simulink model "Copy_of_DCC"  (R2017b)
settings: Solver=FixedStepDiscrete  StartTime=0.0  StopTime=10.0  FixedStep=0.01  RelTol=1e-3  EnableMultiTasking=on
undefined symbols (not defined in the file): ASWTYPE_FALSE, ASWTYPE_TRUE, CbDCC_BMTMsgCmd_flg, CbDCC_BMVMsgCmd_flg, CbDCC_BSPMsgCmd_flg, CcDCC_BSTSendTi_ms, CcDCC_BulkSOC_pct, CcDCC_CCSTout_ms, CcDCC_CellTempFilterAvg_numb, CcDCC_ChrgCrnt0HysVolt_mV, CcDCC_ChrgFinOverTi_ms, CcDCC_ChrgMaxPackVoltLimt_V, CcDCC_ChrgSt2StepChrgTime_ms, CcDCC_ChrgStCutoffTime_ms, CcDCC_ChrgStFullChrgCrnt_A, CcDCC_CMLTout_ms, CcDCC_CommToutOverTi_ms, CcDCC_CRMAATout_ms, CcDCC_CRMCHMTout_ms, CcDCC_CRMTout_ms, CcDCC_CROAATout_ms, CcDCC_CROTout_ms, CcDCC_CSDTout_ms, CcDCC_CSTTout_ms, CcDCC_DC12VUnonnectTi_ms, CcDCC_DCChrgDispSOCPrmt_pct, CcDCC_DCChrgMismatch_ms, CcDCC_DCChrgPermitCfg_ms, CcDCC_DCChrgPrmtFltLvl_numb, CcDCC_DCChrgPrmtStop_ms, CcDCC_DCChrgStepCurr_A, CcDCC_DCChrgStop_ms, CcDCC_DCCrntUnctrolTi_ms, CcDCC_DCFullChrgHysVolt_mV, CcDCC_DCFullStepChrgTi1_ms, CcDCC_DCFullStepChrgTi2_ms, CcDCC_DCMaxChrgCurr_A, CcDCC_DCStepChrgWaitTime_ms, CcDCC_DCStop2DefaultTi_ms, CcDCC_DefaultWaitTi_ms, CcDCC_DiffDCChrgCrnt_A, CcDCC_DiffDCChrgCrntTi_ms, CcDCC_HeatChrgCrnt0Time_ms, CcDCC_HeatChrgCrnt1Time_ms, CcDCC_IsoDisableDelay_ms, CcDCC_MaxPackVoltLimt_V, CcDCC_SafeCur_A, CcDCC_StartChrgHysVolt_mV, CcDCC_StartDCChrgCellTemp_C, CcDCC_StepChrgCutoffTi_ms, CcDCC_StepChrgFullChrgCrnt_A, CcDCC_ToutDelay_ms, CcDCC_VehSpdFld_kmh, DCC_CONST0_NUMB, DCC_CONST1000_NUMB, DCC_CONST170_NUMB, DCC_RUNTIME_MS, Enum_BTMHeatReq, Enum_CTCCtrCtlConnMode, Enum_CTCCtrCtlState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
libraries: AIWAYS_Powertrain_BMS_lib x82
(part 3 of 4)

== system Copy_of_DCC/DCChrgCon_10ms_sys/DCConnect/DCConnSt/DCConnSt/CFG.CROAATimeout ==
  GbGDP_CRORecOnce_flg : Inport  OutDataTypeStr=boolean
  GbDCC_BROMsgCmd_flg : Inport  Port=2  OutDataTypeStr=boolean
  GcGDP_CROChrgrRdy_numb : Inport  Port=3  OutDataTypeStr=uint8
  GcDCS_2829Da_numb : Inport  Port=4  OutDataTypeStr=uint8
  CROAATimeout : TriggerPort  TriggerType=function-call  VariantControl=(inherit)  StatesWhenEnabling=reset
  Constant10 : Constant  Value=CcDCC_CROAATout_ms
  Constant11 : Constant  Value=DCC_CONST170_NUMB
  Constant12 : Constant  Value=DCC_CONST170_NUMB
  Constant8 : Constant  Value=ASWTYPE_TRUE
  Constant9 : Constant  Value=DCC_RUNTIME_MS
  Delay2 : AIWAYS_Powertrain_BMS_lib/Debounce & Delay/BMSDelay
  Logical Operator2 : Logic  Inputs=4  AllPortsSameDT=off  OutDataTypeStr=boolean
  Relational Operator3 : RelationalOperator  Operator===  OutDataTypeStr=boolean
  Relational Operator4 : RelationalOperator  Operator===  OutDataTypeStr=boolean
  Relational Operator5 : RelationalOperator  Operator=~=  OutDataTypeStr=boolean
  GbDCC_CROAATout_flg : Outport  OutDataTypeStr=boolean
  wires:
  GcDCS_2829Da_numb/1 -> Relational Operator4/1
  GcGDP_CROChrgrRdy_numb/1 -> Relational Operator5/1
  GbDCC_BROMsgCmd_flg/1 -> Logical Operator2/2
  GbGDP_CRORecOnce_flg/1 -> Relational Operator3/1
  Constant9/1 -> Delay2/2
  Constant11/1 -> Relational Operator5/2
  Constant12/1 -> Relational Operator4/2
  Constant10/1 -> Delay2/3
  Delay2/1 -> Logical Operator2/4
  Relational Operator5/1 -> Logical Operator2/3
  Constant8/1 -> Relational Operator3/2
  Relational Operator4/1 -> Delay2/1
  Relational Operator3/1 -> Logical Operator2/1
  Logical Operator2/1 -> GbDCC_CROAATout_flg/1

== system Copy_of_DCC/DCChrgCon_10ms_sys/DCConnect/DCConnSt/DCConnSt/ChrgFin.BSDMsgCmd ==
  GbGDP_CSTRecOnce_flg : Inport  OutDataTypeStr=boolean
  GbDCC_CSTTout_flg : Inport  Port=2
  BSDMsgCmd : TriggerPort  TriggerType=function-call  VariantControl=(inherit)  StatesWhenEnabling=reset
  Constant2 : Constant  Value=DCC_RUNTIME_MS
  Constant3 : Constant  Value=CcDCC_BSTSendTi_ms
  Delay : AIWAYS_Powertrain_BMS_lib/Debounce & Delay/BMSDelay
  Logical Operator : Logic  Operator=OR  AllPortsSameDT=off  OutDataTypeStr=boolean
  GbDCC_BSDMsgCmd_flg : Outport  OutDataTypeStr=boolean
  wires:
  Logical Operator/1 -> GbDCC_BSDMsgCmd_flg/1
  GbDCC_CSTTout_flg/1 -> Logical Operator/2
  Delay/1 -> Logical Operator/1
  Constant2/1 -> Delay/2
  Constant3/1 -> Delay/3
  GbGDP_CSTRecOnce_flg/1 -> Delay/1

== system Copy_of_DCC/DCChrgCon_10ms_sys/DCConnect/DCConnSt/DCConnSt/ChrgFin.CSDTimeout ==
  GbGDP_CSDRecOnce_flg : Inport  OutDataTypeStr=boolean
  CSDTimeout : TriggerPort  TriggerType=function-call  VariantControl=(inherit)  StatesWhenEnabling=reset
  Constant : Constant  Value=ASWTYPE_TRUE
  Constant2 : Constant  Value=DCC_RUNTIME_MS
  Constant3 : Constant  Value=CcDCC_CSDTout_ms
  Constant4 : Constant  Value=ASWTYPE_FALSE
  Delay : AIWAYS_Powertrain_BMS_lib/Debounce & Delay/BMSDelay
  Logical Operator : Logic  AllPortsSameDT=off  OutDataTypeStr=boolean
  Relational Operator1 : RelationalOperator  Operator===  OutDataTypeStr=boolean
  GbDCC_CSDTout_flg : Outport  OutDataTypeStr=boolean
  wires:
  Logical Operator/1 -> GbDCC_CSDTout_flg/1
  GbGDP_CSDRecOnce_flg/1 -> Relational Operator1/1
  Constant2/1 -> Delay/2
  Constant3/1 -> Delay/3
  Relational Operator1/1 -> Logical Operator/1
  Constant/1 -> Delay/1
  Delay/1 -> Logical Operator/2
  Constant4/1 -> Relational Operator1/2

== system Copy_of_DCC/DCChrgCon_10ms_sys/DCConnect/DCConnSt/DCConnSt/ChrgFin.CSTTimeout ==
  GbGDP_CSTRecOnce_flg : Inport  OutDataTypeStr=boolean
  CSTTimeout : TriggerPort  TriggerType=function-call  VariantControl=(inherit)  StatesWhenEnabling=reset
  Constant : Constant  Value=ASWTYPE_TRUE
  Constant2 : Constant  Value=DCC_RUNTIME_MS
  Constant3 : Constant  Value=CcDCC_CSTTout_ms
  Constant4 : Constant  Value=ASWTYPE_FALSE
  Delay : AIWAYS_Powertrain_BMS_lib/Debounce & Delay/BMSDelay
  Logical Operator : Logic  AllPortsSameDT=off  OutDataTypeStr=boolean
  Relational Operator1 : RelationalOperator  Operator===  OutDataTypeStr=boolean
  GbDCC_CSTTout_flg : Outport  OutDataTypeStr=boolean
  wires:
  Logical Operator/1 -> GbDCC_CSTTout_flg/1
  Constant4/1 -> Relational Operator1/2
  Constant3/1 -> Delay/3
  Constant2/1 -> Delay/2
  Constant/1 -> Delay/1
  Delay/1 -> Logical Operator/2
  Relational Operator1/1 -> Logical Operator/1
  GbGDP_CSTRecOnce_flg/1 -> Relational Operator1/1

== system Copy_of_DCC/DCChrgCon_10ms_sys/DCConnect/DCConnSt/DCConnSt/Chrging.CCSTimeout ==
  GbGDP_CCSMsgUpd_flg : Inport  OutDataTypeStr=boolean
  CCSTimeout : TriggerPort  TriggerType=function-call  VariantControl=(inherit)  StatesWhenEnabling=reset
  Constant2 : Constant  Value=DCC_RUNTIME_MS
  Constant3 : Constant  Value=CcDCC_CCSTout_ms
  Constant4 : Constant  Value=ASWTYPE_FALSE
  Delay : AIWAYS_Powertrain_BMS_lib/Debounce & Delay/BMSDelay
  Relational Operator : RelationalOperator  Operator===  OutDataTypeStr=boolean
  GbDCC_CCSTout_flg : Outport  OutDataTypeStr=boolean
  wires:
  Delay/1 -> GbDCC_CCSTout_flg/1
  Constant2/1 -> Delay/2
  GbGDP_CCSMsgUpd_flg/1 -> Relational Operator/1
  Constant4/1 -> Relational Operator/2
  Relational Operator/1 -> Delay/1
  Constant3/1 -> Delay/3

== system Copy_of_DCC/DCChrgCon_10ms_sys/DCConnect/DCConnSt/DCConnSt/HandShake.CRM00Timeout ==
  GbGDP_CHMRecOnce_flg : Inport  OutDataTypeStr=boolean
  CRM00Timeout : TriggerPort  TriggerType=function-call  VariantControl=(inherit)  StatesWhenEnabling=reset
  Constant : Constant  Value=ASWTYPE_TRUE
  Constant2 : Constant  Value=DCC_RUNTIME_MS
  Constant3 : Constant  Value=CcDCC_CRMTout_ms
  Constant5 : Constant  Value=DCC_RUNTIME_MS
  Constant6 : Constant  Value=CcDCC_CRMCHMTout_ms
  Constant7 : Constant  Value=ASWTYPE_TRUE
  Delay : AIWAYS_Powertrain_BMS_lib/Debounce & Delay/BMSDelay
  Delay1 : AIWAYS_Powertrain_BMS_lib/Debounce & Delay/BMSDelay
  Logical Operator2 : Logic  Operator=OR  AllPortsSameDT=off  OutDataTypeStr=boolean
  Relational Operator1 : RelationalOperator  Operator===  OutDataTypeStr=boolean
  GbDCC_CRM00Tout_flg : Outport  OutDataTypeStr=boolean
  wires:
  Delay/1 -> Logical Operator2/1
  Constant3/1 -> Delay/3
  Constant/1 -> Delay/1
  Constant2/1 -> Delay/2
  Constant7/1 -> Relational Operator1/2
  Constant6/1 -> Delay1/3
  GbGDP_CHMRecOnce_flg/1 -> Relational Operator1/1
  Constant5/1 -> Delay1/2
  Relational Operator1/1 -> Delay1/1
  Logical Operator2/1 -> GbDCC_CRM00Tout_flg/1
  Delay1/1 -> Logical Operator2/2

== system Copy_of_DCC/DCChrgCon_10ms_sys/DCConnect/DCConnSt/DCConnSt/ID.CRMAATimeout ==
  GbGDP_CRMRecOnce_flg : Inport  OutDataTypeStr=boolean
  GcGDP_CRMChrgrAck_numb : Inport  Port=2  OutDataTypeStr=uint8
  CRMAATimeout : TriggerPort  TriggerType=function-call  VariantControl=(inherit)  StatesWhenEnabling=reset
  Constant : Constant  Value=ASWTYPE_TRUE
  Constant1 : Constant  Value=ASWTYPE_TRUE
  Constant2 : Constant  Value=DCC_RUNTIME_MS
  Constant3 : Constant  Value=CcDCC_CRMAATout_ms
  Constant6 : Constant  Value=DCC_CONST170_NUMB
  Delay : AIWAYS_Powertrain_BMS_lib/Debounce & Delay/BMSDelay
  Logical Operator : Logic  Inputs=3  AllPortsSameDT=off  OutDataTypeStr=boolean
  Relational Operator : RelationalOperator  Operator===  OutDataTypeStr=boolean
  Relational Operator1 : RelationalOperator  Operator=~=  OutDataTypeStr=boolean
  GbDCC_CRMAATout_flg : Outport  OutDataTypeStr=boolean
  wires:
  Logical Operator/1 -> GbDCC_CRMAATout_flg/1
  Delay/1 -> Logical Operator/3
  Constant6/1 -> Relational Operator1/2
  Constant3/1 -> Delay/3
  Constant1/1 -> Relational Operator/2
  Relational Operator1/1 -> Logical Operator/2
  Relational Operator/1 -> Logical Operator/1
  GcGDP_CRMChrgrAck_numb/1 -> Relational Operator1/1
  Constant2/1 -> Delay/2
  GbGDP_CRMRecOnce_flg/1 -> Relational Operator/1
  Constant/1 -> Delay/1

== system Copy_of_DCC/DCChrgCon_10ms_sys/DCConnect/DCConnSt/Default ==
  GeLDP_CC2St_enum : Inport
  GbLDP_DC12VSply_flg : Inport  Port=2
  GcADP_VehSpd_kmh : Inport  Port=3
  Enable : EnablePort  StatesWhenEnabling=reset
  Constant : Constant  Value=Enum_LDPCC2St.Enum_LDPCC2St_Connect
  Constant1 : Constant  Value=ASWTYPE_TRUE
  Constant10 : Constant  Value=CcDCC_DefaultWaitTi_ms
  Constant5 : Constant  Value=CcDCC_VehSpdFld_kmh
  Constant9 : Constant  Value=DCC_RUNTIME_MS
  Data Type Conversion2 : DataTypeConversion
  Delay : AIWAYS_Powertrain_BMS_lib/Debounce & Delay/BMSDelay
  Logical Operator : Logic  Inputs=3  AllPortsSameDT=off  OutDataTypeStr=boolean
  Relational Operator1 : RelationalOperator  Operator===  OutDataTypeStr=boolean
  Relational Operator5 : RelationalOperator  Operator=<  OutDataTypeStr=boolean
  Relational Operator6 : RelationalOperator  Operator===  OutDataTypeStr=boolean
  LbDCC_DCDefault2Handshake_flg : Outport
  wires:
  Constant10/1 -> Delay/3
  Constant9/1 -> Delay/2
  Data Type Conversion2/1 -> Relational Operator6/1
  Constant/1 -> Relational Operator6/2
  GeLDP_CC2St_enum/1 -> Data Type Conversion2/1
  GbLDP_DC12VSply_flg/1 -> Relational Operator1/1
  Relational Operator5/1 -> Logical Operator/3
  Constant5/1 -> Relational Operator5/2
  GcADP_VehSpd_kmh/1 -> Relational Operator5/1
  Relational Operator1/1 -> Logical Operator/2
  Constant1/1 -> Relational Operator1/2
  Relational Operator6/1 -> Logical Operator/1
  Logical Operator/1 -> Delay/1
  Delay/1 -> LbDCC_DCDefault2Handshake_flg/1  "LbDCC_DCDefault2Handshake_flg"

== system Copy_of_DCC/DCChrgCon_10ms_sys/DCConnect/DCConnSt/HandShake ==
  GbLDP_DC12VSply_flg : Inport
  Enable : EnablePort  StatesWhenEnabling=reset
  Constant1 : Constant  Value=DCC_RUNTIME_MS
  Constant2 : Constant  Value=ASWTYPE_FALSE
  Constant5 : Constant  Value=CcDCC_DC12VUnonnectTi_ms
  Delay1 : AIWAYS_Powertrain_BMS_lib/Debounce & Delay/BMSDelay
  Relational Operator1 : RelationalOperator  Operator===  OutDataTypeStr=boolean
  LbDCC_DCHandShake2Default_flg : Outport
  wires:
  Constant1/1 -> Delay1/2
  Constant5/1 -> Delay1/3
  Relational Operator1/1 -> Delay1/1
  Delay1/1 -> LbDCC_DCHandShake2Default_flg/1  "LbDCC_DCHandShake2Default_flg"
  GbLDP_DC12VSply_flg/1 -> Relational Operator1/1
  Constant2/1 -> Relational Operator1/2

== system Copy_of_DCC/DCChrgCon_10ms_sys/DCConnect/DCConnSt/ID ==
  GbLDP_DC12VSply_flg : Inport
  Enable : EnablePort  StatesWhenEnabling=reset
  Constant1 : Constant  Value=DCC_RUNTIME_MS
  Constant2 : Constant  Value=ASWTYPE_FALSE
  Constant5 : Constant  Value=CcDCC_DC12VUnonnectTi_ms
  Delay1 : AIWAYS_Powertrain_BMS_lib/Debounce & Delay/BMSDelay
  Relational Operator1 : RelationalOperator  Operator===  OutDataTypeStr=boolean
  LbDCC_DCID2Default_flg : Outport
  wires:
  Constant1/1 -> Delay1/2
  Constant5/1 -> Delay1/3
  Relational Operator1/1 -> Delay1/1
  Delay1/1 -> LbDCC_DCID2Default_flg/1  "LbDCC_DCID2Default_flg"
  GbLDP_DC12VSply_flg/1 -> Relational Operator1/1
  Constant2/1 -> Relational Operator1/2

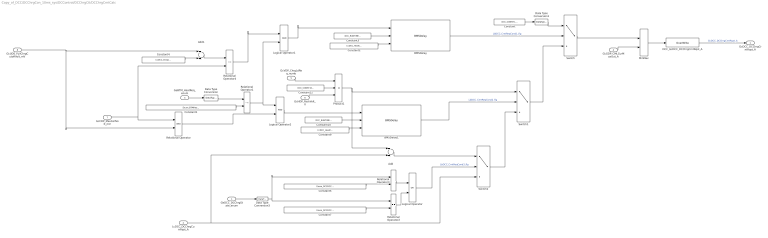
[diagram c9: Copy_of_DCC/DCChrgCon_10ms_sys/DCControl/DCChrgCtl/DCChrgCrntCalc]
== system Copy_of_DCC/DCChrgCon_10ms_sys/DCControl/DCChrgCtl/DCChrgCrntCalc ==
  GeDCC_DCChrgState_enum : Inport
  LcDCC_DCChrgCurrRqst_A : Inport  Port=2
  GeBTM_HeatReq_enum : Inport  Port=3
  GcGDP_CMLCurMaxOut_A : Inport  Port=4
  GcVDP_ChrgLdReq_numb : Inport  Port=5
  GcHDP_PackVolt_V : Inport  Port=6
  GcCDP_MaxCellVolt_mV : Inport  Port=7
  GcUDS_FullChrgCutoffVolt_mV : Inport  Port=8
  Add : Sum  OutDataTypeStr=single
  Add1 : Sum
  BMSDelay : AIWAYS_Powertrain_BMS_lib/Debounce & Delay/BMSDelay
  BMSDelay1 : AIWAYS_Powertrain_BMS_lib/Debounce & Delay/BMSDelay
  Constant : Constant  Value=DCC_CONST0_NUMB
  Constant1 : Constant  Value=Enum_BTMHeatReq.Enum_BTMHeatReq_Default
  Constant10 : Constant  Value=DCC_RUNTIME_MS
  Constant12 : Constant  Value=DCC_CONST1000_NUMB
  Constant2 : Constant  Value=CcDCC_HeatChrgCrnt0Time_ms
  Constant3 : Constant  Value=DCC_RUNTIME_MS
  Constant4 : Constant  Value=CcDCC_ChrgCrnt0HysVolt_mV
  Constant5 : Constant  Value=Enum_DCCDCChrgState.Enum_DCCDCChrgState_Chrg
  Constant7 : Constant  Value=Enum_DCCDCChrgState.Enum_DCCDCChrgState_StepChrg
  Constant9 : Constant  Value=CcDCC_HeatChrgCrnt1Time_ms
  DCC_GcDCC_DCChrgCrntRqst_A : AIWAYS_Powertrain_BMS_lib/Signals/OverWrite  OverWrite_Value=CcDCC_DCChrgCrntRqstOvr_A  OverWrite_flag=CbDCC_DCChrgCrntRqstOvrSwt_flg
  Data Type Conversion : DataTypeConversion
  Data Type Conversion1 : DataTypeConversion
  Data Type Conversion3 : DataTypeConversion
  Logical Operator : Logic  Operator=OR  AllPortsSameDT=off  OutDataTypeStr=boolean
  Logical Operator1 : Logic  AllPortsSameDT=off  OutDataTypeStr=boolean
  Logical Operator2 : Logic  AllPortsSameDT=off  OutDataTypeStr=boolean
  MinMax : MinMax  Inputs=2
  Product1 : Product  Inputs=**/  OutDataTypeStr=Inherit: Inherit via back propagation
  Relational Operator : RelationalOperator  OutDataTypeStr=boolean
  Relational Operator1 : RelationalOperator  Operator=~=  OutDataTypeStr=boolean
  Relational Operator2 : RelationalOperator  Operator===  OutDataTypeStr=boolean
  Relational Operator3 : RelationalOperator  Operator===  OutDataTypeStr=boolean
  Relational Operator4 : RelationalOperator  Operator=<=  OutDataTypeStr=boolean
  Switch : Switch  Criteria=u2 ~= 0  Threshold=1  RndMeth=Zero
  Switch1 : Switch  Criteria=u2 ~= 0  Threshold=1  RndMeth=Zero
  Switch2 : Switch  Criteria=u2 ~= 0  Threshold=1  RndMeth=Zero
  GcDCC_DCChrgCrntRqst_A : Outport
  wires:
  GcGDP_CMLCurMaxOut_A/1 -> MinMax/2
  Relational Operator2/1 -> Logical Operator/2
  Constant7/1 -> Relational Operator2/2
  Constant5/1 -> Relational Operator3/2
  Relational Operator3/1 -> Logical Operator/1
  GeDCC_DCChrgState_enum/1 -> Data Type Conversion3/1
  LcDCC_DCChrgCurrRqst_A/1 -> Add/2, Switch2/3
  Data Type Conversion3/1 -> Relational Operator3/1, Relational Operator2/1
  GcVDP_ChrgLdReq_numb/1 -> Product1/1
  Constant1/1 -> Relational Operator1/2
  GeBTM_HeatReq_enum/1 -> Data Type Conversion/1
  GcCDP_MaxCellVolt_mV/1 -> Relational Operator4/2, Relational Operator/1
  Constant2/1 -> BMSDelay/3
  Constant3/1 -> BMSDelay/2
  GcUDS_FullChrgCutoffVolt_mV/1 -> Relational Operator/2, Add1/1
  Constant4/1 -> Add1/2
  Add1/1 -> Relational Operator4/1
  Data Type Conversion/1 -> Relational Operator1/1
  Relational Operator4/1 -> Logical Operator1/1
  Relational Operator1/1 -> Logical Operator2/1, Logical Operator1/2
  Relational Operator/1 -> Logical Operator2/2
  Logical Operator1/1 -> BMSDelay/1
  Logical Operator2/1 -> BMSDelay1/1
  Constant10/1 -> BMSDelay1/2
  Constant9/1 -> BMSDelay1/3
  BMSDelay/1 -> Switch/2  "LbDCC_CrntReqCond1_flg"
  Constant/1 -> Data Type Conversion1/1
  BMSDelay1/1 -> Switch1/2  "LbDCC_CrntReqCond2_flg"
  Switch1/1 -> Switch/3
  Product1/1 -> Add/1, Switch1/1
  Logical Operator/1 -> Switch2/2  "LbDCC_CrntReqCond3_flg"
  Switch2/1 -> Switch1/3
  Add/1 -> Switch2/1
  GcHDP_PackVolt_V/1 -> Product1/3
  Constant12/1 -> Product1/2
  Switch/1 -> MinMax/1
  MinMax/1 -> DCC_GcDCC_DCChrgCrntRqst_A/1
  DCC_GcDCC_DCChrgCrntRqst_A/1 -> GcDCC_DCChrgCrntRqst_A/1  "GcDCC_DCChrgCrntRqst_A"
  Data Type Conversion1/1 -> Switch/1

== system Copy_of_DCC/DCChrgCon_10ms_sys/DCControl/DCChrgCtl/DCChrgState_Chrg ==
  GcDCC_DCChrgCrntRqst_A : Inport
  GcCDP_MaxCellVolt_mV : Inport  Port=2
  GeBTM_HeatReq_enum : Inport  Port=3
  GbDCC_DCChrgPrmt_flg : Inport  Port=4
  GeVDP_ChrgRqst_enum : Inport  Port=5
  GeDCC_DCConnSt_enum : Inport  Port=6
  GcUDS_FullChrgCutoffVolt_mV : Inport  Port=7
  Enable : EnablePort  StatesWhenEnabling=reset
  Bus Creator : BusCreator  Inputs=7
  Bus Selector : BusSelector  OutputSignals=GcDCC_DCChrgCrntRqst_A,GcCDP_MaxCellVolt_mV,GeBTM_HeatReq_enum,GcUDS_FullChrgCutoffVolt_mV
  Bus Selector1 : BusSelector  OutputSignals=GbDCC_DCChrgPrmt_flg,GcDCC_DCChrgCrntRqst_A,GcCDP_MaxCellVolt_mV,GeBTM_HeatReq_enum,GeVDP_ChrgRqst_enum,GeDCC_DCConnSt_enum,GcUDS_FullChrgCutoffVolt_mV
  Bus Selector2 : BusSelector  OutputSignals=GcCDP_MaxCellVolt_mV,GcUDS_FullChrgCutoffVolt_mV
  DCChrgCrntUnctrol : Subsystem
  DCChrgStateChrg2StepChrg : Subsystem
  DCChrgStateChrg2Stop : Subsystem
  LbDCC_ChrgSt2StepChrg_flg : Outport
  LbDCC_ChrgSt2Stop_flg : Outport  Port=2
  LbDCC_FinishInChrgSt_flg : Outport  Port=3
  GbDCC_DCCrntUnctrolFlt_flg : Outport  Port=4
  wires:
  DCChrgStateChrg2StepChrg/1(LbDCC_ChrgSt2StepChrg_flg) -> LbDCC_ChrgSt2StepChrg_flg/1
  DCChrgStateChrg2Stop/1(LbDCC_ChrgSt2Stop_flg) -> LbDCC_ChrgSt2Stop_flg/1
  DCChrgStateChrg2Stop/2(LbDCC_FinishInChrgSt_flg) -> LbDCC_FinishInChrgSt_flg/1
  GcDCC_DCChrgCrntRqst_A/1 -> Bus Creator/1
  GcCDP_MaxCellVolt_mV/1 -> Bus Creator/2
  GeBTM_HeatReq_enum/1 -> Bus Creator/3
  GbDCC_DCChrgPrmt_flg/1 -> Bus Creator/4
  GeVDP_ChrgRqst_enum/1 -> Bus Creator/5
  Bus Creator/1 -> Bus Selector/1, Bus Selector1/1, Bus Selector2/1
  Bus Selector/1 -> DCChrgStateChrg2StepChrg/1(GcDCC_DCChrgCrntRqst_A)  "<GcDCC_DCChrgCrntRqst_A>"
  Bus Selector/2 -> DCChrgStateChrg2StepChrg/2(GcCDP_MaxCellVolt_mV)  "<GcCDP_MaxCellVolt_mV>"
  Bus Selector/3 -> DCChrgStateChrg2StepChrg/3(GeBTM_HeatReq_enum)  "<GeBTM_HeatReq_enum>"
  Bus Selector1/1 -> DCChrgStateChrg2Stop/1(GbDCC_DCChrgPrmt_flg)  "<GbDCC_DCChrgPrmt_flg>"
  Bus Selector1/2 -> DCChrgStateChrg2Stop/2(GcDCC_DCChrgCrntRqst_A)  "<GcDCC_DCChrgCrntRqst_A>"
  Bus Selector1/3 -> DCChrgStateChrg2Stop/3(GcCDP_MaxCellVolt_mV)  "<GcCDP_MaxCellVolt_mV>"
  Bus Selector1/4 -> DCChrgStateChrg2Stop/4(GeBTM_HeatReq_enum)  "<GeBTM_HeatReq_enum>"
  DCChrgCrntUnctrol/1(GbDCC_DCCrntUnctrolFlt_flg) -> DCChrgStateChrg2Stop/8(GbDCC_DCCrntUnctrolFlt_flg), GbDCC_DCCrntUnctrolFlt_flg/1
  Bus Selector1/5 -> DCChrgStateChrg2Stop/5(GeVDP_ChrgRqst_enum)  "<GeVDP_ChrgRqst_enum>"
  Bus Selector2/1 -> DCChrgCrntUnctrol/1(GcCDP_MaxCellVolt_mV)  "<GcCDP_MaxCellVolt_mV>"
  GeDCC_DCConnSt_enum/1 -> Bus Creator/6
  Bus Selector1/6 -> DCChrgStateChrg2Stop/6(GeDCC_DCConnSt_enum)  "<GeDCC_DCConnSt_enum>"
  GcUDS_FullChrgCutoffVolt_mV/1 -> Bus Creator/7
  Bus Selector/4 -> DCChrgStateChrg2StepChrg/4(GcUDS_FullChrgCutoffVolt_mV)  "<GcUDS_FullChrgCutoffVolt_mV>"
  Bus Selector2/2 -> DCChrgCrntUnctrol/2(GcUDS_FullChrgCutoffVolt_mV)  "<GcUDS_FullChrgCutoffVolt_mV>"
  Bus Selector1/7 -> DCChrgStateChrg2Stop/7(GcUDS_FullChrgCutoffVolt_mV)  "<GcUDS_FullChrgCutoffVolt_mV>"

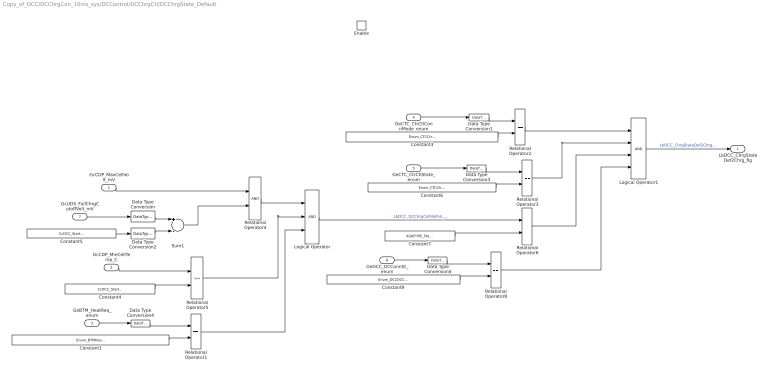
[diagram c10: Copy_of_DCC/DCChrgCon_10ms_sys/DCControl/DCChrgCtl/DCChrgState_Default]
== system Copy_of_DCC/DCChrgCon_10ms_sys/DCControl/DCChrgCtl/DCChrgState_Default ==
  GcCDP_MaxCellVolt_mV : Inport
  GcCDP_MinCellTemp_C : Inport  Port=2
  GeBTM_HeatReq_enum : Inport  Port=3
  GeCTC_CtrCtlConnMode_enum : Inport  Port=4
  GeCTC_CtrCtlState_enum : Inport  Port=5
  GeDCC_DCConnSt_enum : Inport  Port=6
  GcUDS_FullChrgCutoffVolt_mV : Inport  Port=7
  Enable : EnablePort  StatesWhenEnabling=reset
  Constant1 : Constant  Value=Enum_BTMHeatReq.Enum_BTMHeatReq_Default
  Constant3 : Constant  Value=Enum_CTCCtrCtlConnMode.Enum_CTCCtrCtlConnMode_DCChrg
  Constant4 : Constant  Value=CcDCC_StartDCChrgCellTemp_C
  Constant5 : Constant  Value=CcDCC_StartChrgHysVolt_mV
  Constant6 : Constant  Value=Enum_CTCCtrCtlState.Enum_CTCCtrCtlState_Online
  Constant7 : Constant  Value=ASWTYPE_FALSE
  Constant9 : Constant  Value=Enum_DCCDCConnSt.Enum_DCCDCConnSt_Chrging
  Data Type Conversion : DataTypeConversion  OutDataTypeStr=single
  Data Type Conversion{1,3..5} (4 alike) : DataTypeConversion
  Data Type Conversion2 : DataTypeConversion  OutDataTypeStr=single
  Logical Operator : Logic  Inputs=3  AllPortsSameDT=off  OutDataTypeStr=boolean
  Logical Operator1 : Logic  Inputs=4  AllPortsSameDT=off  OutDataTypeStr=boolean
  Relational Operator{1..3,6,8} (5 alike) : RelationalOperator  Operator===  OutDataTypeStr=boolean
  Relational Operator4 : RelationalOperator  OutDataTypeStr=boolean
  Relational Operator5 : RelationalOperator  Operator=<=  OutDataTypeStr=boolean
  Sum1 : Sum  Inputs=+-  OutDataTypeStr=Inherit: Inherit via back propagation  RndMeth=Zero
  LbDCC_ChrgStateDef2Chrg_flg : Outport
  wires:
  GcCDP_MaxCellVolt_mV/1 -> Relational Operator4/1
  Logical Operator/1 -> Relational Operator6/1  "LbDCC_DCChrgCellVoltHi_flg"
  Relational Operator4/1 -> Logical Operator/1
  Relational Operator5/1 -> Logical Operator/2
  Constant1/1 -> Relational Operator1/2
  GeBTM_HeatReq_enum/1 -> Data Type Conversion4/1
  Data Type Conversion4/1 -> Relational Operator1/1
  GcCDP_MinCellTemp_C/1 -> Relational Operator5/1
  GcUDS_FullChrgCutoffVolt_mV/1 -> Data Type Conversion/1
  Constant4/1 -> Relational Operator5/2
  Sum1/1 -> Relational Operator4/2
  Relational Operator1/1 -> Logical Operator/3
  Constant5/1 -> Data Type Conversion2/1
  GeCTC_CtrCtlConnMode_enum/1 -> Data Type Conversion1/1
  Logical Operator1/1 -> LbDCC_ChrgStateDef2Chrg_flg/1  "LbDCC_ChrgStateDef2Chrg_flg"
  Constant7/1 -> Relational Operator6/2
  Relational Operator6/1 -> Logical Operator1/3
  Relational Operator3/1 -> Logical Operator1/2
  Constant3/1 -> Relational Operator2/2
  Data Type Conversion3/1 -> Relational Operator3/1
  Data Type Conversion1/1 -> Relational Operator2/1
  Constant6/1 -> Relational Operator3/2
  GeCTC_CtrCtlState_enum/1 -> Data Type Conversion3/1
  Data Type Conversion/1 -> Sum1/1
  Data Type Conversion2/1 -> Sum1/2
  Relational Operator2/1 -> Logical Operator1/1
  Constant9/1 -> Relational Operator8/2
  GeDCC_DCConnSt_enum/1 -> Data Type Conversion5/1
  Data Type Conversion5/1 -> Relational Operator8/1
  Relational Operator8/1 -> Logical Operator1/4

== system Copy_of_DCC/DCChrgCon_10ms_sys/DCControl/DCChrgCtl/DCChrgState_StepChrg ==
  GcDCC_DCChrgCrntRqst_A : Inport
  GcCDP_MaxCellVolt_mV : Inport  Port=2
  GbDCC_DCChrgPrmt_flg : Inport  Port=3
  GeVDP_ChrgRqst_enum : Inport  Port=4
  GeDCC_DCConnSt_enum : Inport  Port=5
  GcUDS_FullChrgCutoffVolt_mV : Inport  Port=6
  Enable : EnablePort  StatesWhenEnabling=reset
  DCCrntInStepChrgRequest : Subsystem
  DCCurrentDecrease : Subsystem
  DCFullChrg : Subsystem
  DCStepChrg2Stop : Subsystem
  LcDCC_StepChrgCrntReq_A : Outport
  LbDCC_StepChrg2Stop_flg : Outport  Port=2
  LbDCC_FinishInStepChrg_flg : Outport  Port=3
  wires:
  GcDCC_DCChrgCrntRqst_A/1 -> DCCurrentDecrease/1(GcDCC_DCChrgCrntRqst_A)
  GcCDP_MaxCellVolt_mV/1 -> DCFullChrg/3(GcCDP_MaxCellVolt_mV), DCCurrentDecrease/2(GcCDP_MaxCellVolt_mV)
  GbDCC_DCChrgPrmt_flg/1 -> DCStepChrg2Stop/2(GbDCC_DCChrgPrmt_flg)
  DCCurrentDecrease/1(LbDCC_StepChrgVoltReach_flg) -> DCCrntInStepChrgRequest/1(LbDCC_StepChrgVoltReach_flg)
  DCCurrentDecrease/2(LcDCC_StepChrgCrntDec_A) -> DCCrntInStepChrgRequest/2(LcDCC_StepChrgCrntDec_A)
  DCCrntInStepChrgRequest/1(LcDCC_StepChrgCrntReq_A) -> DCFullChrg/1(LcDCC_StepChrgCrntReq_A), LcDCC_StepChrgCrntReq_A/1
  DCFullChrg/1(LbDCC_FinishInStepChrg_flg) -> LbDCC_FinishInStepChrg_flg/1, DCStepChrg2Stop/1(LbDCC_FinishInStepChrg_flg)
  DCStepChrg2Stop/1(LbDCC_StepChrg2Stop_flg) -> LbDCC_StepChrg2Stop_flg/1
  GeVDP_ChrgRqst_enum/1 -> DCStepChrg2Stop/3(GeVDP_ChrgRqst_enum)
  GeDCC_DCConnSt_enum/1 -> DCStepChrg2Stop/4(GeDCC_DCConnSt_enum)
  GcUDS_FullChrgCutoffVolt_mV/1 -> DCCurrentDecrease/3(GcUDS_FullChrgCutoffVolt_mV), DCFullChrg/2(GcUDS_FullChrgCutoffVolt_mV)

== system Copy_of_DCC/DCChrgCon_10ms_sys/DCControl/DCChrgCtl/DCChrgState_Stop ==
  GeDCC_DCConnSt_enum : Inport
  Enable : EnablePort  StatesWhenEnabling=reset
  BMSDelay : AIWAYS_Powertrain_BMS_lib/Debounce & Delay/BMSDelay
  Constant : Constant  Value=ASWTYPE_TRUE
  Constant3 : Constant  Value=Enum_DCCDCConnSt.Enum_DCCDCConnSt_ID
  Constant4 : Constant  Value=CcDCC_DCStop2DefaultTi_ms
  Constant5 : Constant  Value=DCC_RUNTIME_MS
  Data Type Conversion5 : DataTypeConversion
  EdgeRising : AIWAYS_Powertrain_BMS_lib/Logical Operators/EdgeRising
  Logical1 : Logic  Operator=OR  OutDataTypeStr=boolean
  Relational Operator8 : RelationalOperator  Operator===  OutDataTypeStr=boolean
  LbDCC_Stop2Default_flg : Outport
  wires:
  Constant4/1 -> BMSDelay/3
  Constant5/1 -> BMSDelay/2
  Constant/1 -> BMSDelay/1
  Data Type Conversion5/1 -> Relational Operator8/1
  Constant3/1 -> Relational Operator8/2
  GeDCC_DCConnSt_enum/1 -> Data Type Conversion5/1
  Relational Operator8/1 -> EdgeRising/1
  BMSDelay/1 -> Logical1/1
  EdgeRising/1 -> Logical1/2
  Logical1/1 -> LbDCC_Stop2Default_flg/1  "LbDCC_Stop2Default_flg"

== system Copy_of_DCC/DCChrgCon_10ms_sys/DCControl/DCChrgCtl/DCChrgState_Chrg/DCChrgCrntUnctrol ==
  GcCDP_MaxCellVolt_mV : Inport
  GcUDS_FullChrgCutoffVolt_mV : Inport  Port=2
  Add : Sum
  BMSDebounceStartZero : AIWAYS_Powertrain_BMS_lib/Debounce & Delay/BMSDebounceStartZero
  Constant10 : Constant  Value=CcDCC_DCFullChrgHysVolt_mV
  Constant2 : Constant  Value=DCC_RUNTIME_MS
  Constant3 : Constant  Value=CcDCC_DCCrntUnctrolTi_ms
  Constant7 : Constant  Value=DCC_RUNTIME_MS
  Constant9 : Constant  Value=CcDCC_DCCrntUnctrolTi_ms
  DCC_GbDCC_DCCrntUnctrolFlt_flg : AIWAYS_Powertrain_BMS_lib/Signals/OverWrite  OverWrite_Value=CbDCC_DCCrntUnctrolFltOvr_flg  OverWrite_flag=CbDCC_DCCrntUnctrolFltOvrSwt_flg
  Relational Operator4 : RelationalOperator  OutDataTypeStr=boolean
  GbDCC_DCCrntUnctrolFlt_flg : Outport
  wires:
  GcCDP_MaxCellVolt_mV/1 -> Relational Operator4/1
  Add/1 -> Relational Operator4/2
  Constant10/1 -> Add/2
  Constant9/1 -> BMSDebounceStartZero/4
  Constant7/1 -> BMSDebounceStartZero/3
  GcUDS_FullChrgCutoffVolt_mV/1 -> Add/1
  Relational Operator4/1 -> BMSDebounceStartZero/1
  BMSDebounceStartZero/1 -> DCC_GbDCC_DCCrntUnctrolFlt_flg/1
  DCC_GbDCC_DCCrntUnctrolFlt_flg/1 -> GbDCC_DCCrntUnctrolFlt_flg/1  "GbDCC_DCCrntUnctrolFlt_flg"
  Constant2/1 -> BMSDebounceStartZero/5
  Constant3/1 -> BMSDebounceStartZero/2

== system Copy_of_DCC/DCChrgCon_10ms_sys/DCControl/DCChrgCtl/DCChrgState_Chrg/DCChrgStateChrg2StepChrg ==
  GcDCC_DCChrgCrntRqst_A : Inport
  GcCDP_MaxCellVolt_mV : Inport  Port=2
  GeBTM_HeatReq_enum : Inport  Port=3
  GcUDS_FullChrgCutoffVolt_mV : Inport  Port=4
  BMSDebounceStartZero : AIWAYS_Powertrain_BMS_lib/Debounce & Delay/BMSDebounceStartZero
  Constant1 : Constant  Value=CcDCC_ChrgSt2StepChrgTime_ms
  Constant2 : Constant  Value=DCC_RUNTIME_MS
  Constant3 : Constant  Value=Enum_BTMHeatReq.Enum_BTMHeatReq_Default
  Constant5 : Constant  Value=CcDCC_ChrgStFullChrgCrnt_A
  Constant6 : Constant  Value=DCC_RUNTIME_MS
  Constant7 : Constant  Value=CcDCC_ChrgSt2StepChrgTime_ms
  Data Type Conversion4 : DataTypeConversion
  Logical Operator : Logic  Inputs=3  AllPortsSameDT=off  OutDataTypeStr=boolean
  Relational Operator : RelationalOperator  OutDataTypeStr=boolean
  Relational Operator1 : RelationalOperator  Operator===  OutDataTypeStr=boolean
  Relational Operator3 : RelationalOperator  Operator=>  OutDataTypeStr=boolean
  LbDCC_ChrgSt2StepChrg_flg : Outport
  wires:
  GcCDP_MaxCellVolt_mV/1 -> Relational Operator/1
  Constant5/1 -> Relational Operator3/2
  Relational Operator3/1 -> Logical Operator/1
  GcUDS_FullChrgCutoffVolt_mV/1 -> Relational Operator/2
  Logical Operator/1 -> BMSDebounceStartZero/1
  Relational Operator/1 -> Logical Operator/2
  GcDCC_DCChrgCrntRqst_A/1 -> Relational Operator3/1
  Relational Operator1/1 -> Logical Operator/3
  Constant3/1 -> Relational Operator1/2
  GeBTM_HeatReq_enum/1 -> Data Type Conversion4/1
  Data Type Conversion4/1 -> Relational Operator1/1
  Constant2/1 -> BMSDebounceStartZero/3
  Constant1/1 -> BMSDebounceStartZero/4
  BMSDebounceStartZero/1 -> LbDCC_ChrgSt2StepChrg_flg/1  "LbDCC_ChrgSt2StepChrg_flg"
  Constant6/1 -> BMSDebounceStartZero/5
  Constant7/1 -> BMSDebounceStartZero/2

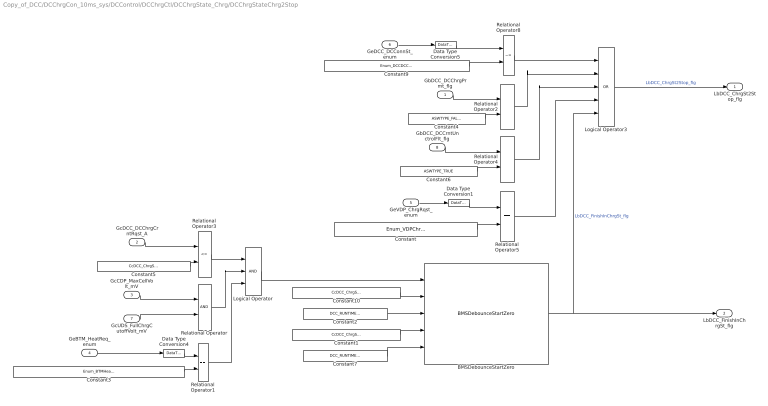
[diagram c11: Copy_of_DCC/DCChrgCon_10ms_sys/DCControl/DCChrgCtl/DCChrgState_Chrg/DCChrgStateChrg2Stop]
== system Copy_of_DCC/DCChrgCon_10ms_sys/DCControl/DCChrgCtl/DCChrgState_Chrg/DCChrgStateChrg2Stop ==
  GbDCC_DCChrgPrmt_flg : Inport
  GcDCC_DCChrgCrntRqst_A : Inport  Port=2
  GcCDP_MaxCellVolt_mV : Inport  Port=3
  GeBTM_HeatReq_enum : Inport  Port=4
  GeVDP_ChrgRqst_enum : Inport  Port=5
  GeDCC_DCConnSt_enum : Inport  Port=6
  GcUDS_FullChrgCutoffVolt_mV : Inport  Port=7
  GbDCC_DCCrntUnctrolFlt_flg : Inport  Port=8
  BMSDebounceStartZero : AIWAYS_Powertrain_BMS_lib/Debounce & Delay/BMSDebounceStartZero
  Constant : Constant  Value=Enum_VDPChrgRqst.Enum_VDPChrgRqst_PowerDown
  Constant1 : Constant  Value=CcDCC_ChrgStCutoffTime_ms
  Constant10 : Constant  Value=CcDCC_ChrgStCutoffTime_ms
  Constant2 : Constant  Value=DCC_RUNTIME_MS
  Constant3 : Constant  Value=Enum_BTMHeatReq.Enum_BTMHeatReq_Default
  Constant4 : Constant  Value=ASWTYPE_FALSE
  Constant5 : Constant  Value=CcDCC_ChrgStFullChrgCrnt_A
  Constant6 : Constant  Value=ASWTYPE_TRUE
  Constant7 : Constant  Value=DCC_RUNTIME_MS
  Constant9 : Constant  Value=Enum_DCCDCConnSt.Enum_DCCDCConnSt_Chrging
  Data Type Conversion1 : DataTypeConversion
  Data Type Conversion4 : DataTypeConversion
  Data Type Conversion5 : DataTypeConversion
  Logical Operator : Logic  Inputs=3  AllPortsSameDT=off  OutDataTypeStr=boolean
  Logical Operator3 : Logic  Operator=OR  Inputs=5  AllPortsSameDT=off  OutDataTypeStr=boolean
  Relational Operator : RelationalOperator  OutDataTypeStr=boolean
  Relational Operator{1..2,4..5} (4 alike) : RelationalOperator  Operator===  OutDataTypeStr=boolean
  Relational Operator3 : RelationalOperator  Operator=<=  OutDataTypeStr=boolean
  Relational Operator8 : RelationalOperator  Operator=~=  OutDataTypeStr=boolean
  LbDCC_ChrgSt2Stop_flg : Outport
  LbDCC_FinishInChrgSt_flg : Outport  Port=2
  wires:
  BMSDebounceStartZero/1 -> Logical Operator3/5, LbDCC_FinishInChrgSt_flg/1  "LbDCC_FinishInChrgSt_flg"
  Logical Operator3/1 -> LbDCC_ChrgSt2Stop_flg/1  "LbDCC_ChrgSt2Stop_flg"
  Constant4/1 -> Relational Operator2/2
  GbDCC_DCChrgPrmt_flg/1 -> Relational Operator2/1
  Constant1/1 -> BMSDebounceStartZero/4
  Constant5/1 -> Relational Operator3/2
  Relational Operator3/1 -> Logical Operator/1
  Logical Operator/1 -> BMSDebounceStartZero/1
  Relational Operator/1 -> Logical Operator/2
  GcDCC_DCChrgCrntRqst_A/1 -> Relational Operator3/1
  Constant3/1 -> Relational Operator1/2
  GeBTM_HeatReq_enum/1 -> Data Type Conversion4/1
  Data Type Conversion4/1 -> Relational Operator1/1
  Constant2/1 -> BMSDebounceStartZero/3
  GcCDP_MaxCellVolt_mV/1 -> Relational Operator/1
  Relational Operator1/1 -> Logical Operator/3
  GcUDS_FullChrgCutoffVolt_mV/1 -> Relational Operator/2
  Constant6/1 -> Relational Operator4/2
  GbDCC_DCCrntUnctrolFlt_flg/1 -> Relational Operator4/1
  Constant/1 -> Relational Operator5/2
  GeVDP_ChrgRqst_enum/1 -> Data Type Conversion1/1
  Data Type Conversion1/1 -> Relational Operator5/1
  GeDCC_DCConnSt_enum/1 -> Data Type Conversion5/1
  Constant9/1 -> Relational Operator8/2
  Data Type Conversion5/1 -> Relational Operator8/1
  Relational Operator8/1 -> Logical Operator3/1
  Relational Operator2/1 -> Logical Operator3/2
  Relational Operator4/1 -> Logical Operator3/3
  Relational Operator5/1 -> Logical Operator3/4
  Constant7/1 -> BMSDebounceStartZero/5
  Constant10/1 -> BMSDebounceStartZero/2

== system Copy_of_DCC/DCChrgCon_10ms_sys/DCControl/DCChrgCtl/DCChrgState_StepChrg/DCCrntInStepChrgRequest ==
  LbDCC_StepChrgVoltReach_flg : Inport  OutDataTypeStr=boolean
  LcDCC_StepChrgCrntDec_A : Inport  Port=2
  Constant : Constant  Value=DCC_CONST0_NUMB
  Data Type Conversion : DataTypeConversion
  Switch : Switch  Criteria=u2 ~= 0
  LcDCC_StepChrgCrntReq_A : Outport
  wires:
  LcDCC_StepChrgCrntDec_A/1 -> Switch/3
  Switch/1 -> LcDCC_StepChrgCrntReq_A/1  "LcDCC_StepChrgCrntReq_A"
  LbDCC_StepChrgVoltReach_flg/1 -> Switch/2
  Constant/1 -> Data Type Conversion/1
  Data Type Conversion/1 -> Switch/1

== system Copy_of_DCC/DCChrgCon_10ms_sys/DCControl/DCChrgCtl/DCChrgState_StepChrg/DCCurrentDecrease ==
  GcDCC_DCChrgCrntRqst_A : Inport
  GcCDP_MaxCellVolt_mV : Inport  Port=2
  GcUDS_FullChrgCutoffVolt_mV : Inport  Port=3
  BMSDebounceStartZero : AIWAYS_Powertrain_BMS_lib/Debounce & Delay/BMSDebounceStartZero
  Constant1 : Constant  Value=CcDCC_StepChrgCutoffTi_ms
  Constant2 : Constant  Value=DCC_RUNTIME_MS
  Constant4 : Constant  Value=ASWTYPE_FALSE
  Constant5 : Constant  Value=ASWTYPE_FALSE
  Constant6 : Constant  Value=DCC_RUNTIME_MS
  Constant7 : Constant  Value=CcDCC_StepChrgCutoffTi_ms
  DCStepChrgVoltReach : Subsystem  TreatAsAtomicUnit=on
  Logical Operator : Logic  Operator=OR  Inputs=3  AllPortsSameDT=off  OutDataTypeStr=boolean
  Relational Operator : RelationalOperator  OutDataTypeStr=boolean
  Subsystem : Subsystem
  Switch : Switch  Criteria=u2 ~= 0  Threshold=""
  Unit Delay : UnitDelay  InitialCondition=ASWTYPE_TRUE  SampleTime=-1  StateName=StateName
  Unit Delay External IC : AIWAYS_Powertrain_BMS_lib/Delay Blocks/Unit Delay External IC
  Unit Delay1 : UnitDelay  InitialCondition=ASWTYPE_FALSE  SampleTime=-1  StateName=StateName
  Unit Delay2 : UnitDelay  InitialCondition=ASWTYPE_FALSE  SampleTime=-1  StateName=StateName
  LbDCC_StepChrgVoltReach_flg : Outport
  LcDCC_StepChrgCrntDec_A : Outport  Port=2
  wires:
  Unit Delay/1 -> Logical Operator/3, Subsystem/Enable
  Switch/1 -> Logical Operator/1
  Unit Delay2/1 -> Switch/3
  Constant5/1 -> Switch/1
  Unit Delay1/1 -> Switch/2
  Logical Operator/1 -> LbDCC_StepChrgVoltReach_flg/1, DCStepChrgVoltReach/Enable, Unit Delay2/1  "LbDCC_StepChrgVoltReach_flg"
  Constant4/1 -> Unit Delay/1
  Relational Operator/1 -> BMSDebounceStartZero/1
  Constant1/1 -> BMSDebounceStartZero/4
  Constant2/1 -> BMSDebounceStartZero/3
  GcCDP_MaxCellVolt_mV/1 -> Relational Operator/1
  GcUDS_FullChrgCutoffVolt_mV/1 -> Relational Operator/2
  DCStepChrgVoltReach/1(LbDCC_DCStepWaitReach_flg) -> Unit Delay1/1
  Unit Delay External IC/1 -> DCStepChrgVoltReach/1(LcDCC_LastCrntRqst_A)  "LcDCC_LastCrntRqst_A"
  DCStepChrgVoltReach/2(LcDCC_StepChrgCrntDec_A) -> LcDCC_StepChrgCrntDec_A/1, Unit Delay External IC/1
  GcDCC_DCChrgCrntRqst_A/1 -> Subsystem/1(GcDCC_DCChrgCrntRqst_A)
  Subsystem/1(LcDCC_DCChrgCrntRqstLock_A) -> Unit Delay External IC/2
  BMSDebounceStartZero/1 -> Logical Operator/2
  Constant6/1 -> BMSDebounceStartZero/5
  Constant7/1 -> BMSDebounceStartZero/2

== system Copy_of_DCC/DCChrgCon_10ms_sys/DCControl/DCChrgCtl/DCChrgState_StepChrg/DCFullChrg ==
  LcDCC_StepChrgCrntReq_A : Inport
  GcUDS_FullChrgCutoffVolt_mV : Inport  Port=2
  GcCDP_MaxCellVolt_mV : Inport  Port=3
  Add : Sum
  BMSDebounceStartZero : AIWAYS_Powertrain_BMS_lib/Debounce & Delay/BMSDebounceStartZero
  BMSDebounceStartZero1 : AIWAYS_Powertrain_BMS_lib/Debounce & Delay/BMSDebounceStartZero
  Constant : Constant  Value=CcDCC_StepChrgFullChrgCrnt_A
  Constant1 : Constant  Value=CcDCC_DCFullStepChrgTi1_ms
  Constant{2,6,8,10} (4 alike) : Constant  Value=DCC_RUNTIME_MS
  Constant11 : Constant  Value=CcDCC_DCFullStepChrgTi2_ms
  Constant3 : Constant  Value=CcDCC_DCFullChrgHysVolt_mV
  Constant7 : Constant  Value=CcDCC_DCFullStepChrgTi2_ms
  Constant9 : Constant  Value=CcDCC_DCFullStepChrgTi1_ms
  Logical Operator1 : Logic  Operator=OR  AllPortsSameDT=off  OutDataTypeStr=boolean
  Logical Operator2 : Logic  AllPortsSameDT=off  OutDataTypeStr=boolean
  Relational Operator : RelationalOperator  Operator=<=  OutDataTypeStr=boolean
  Relational Operator1 : RelationalOperator  OutDataTypeStr=boolean
  Relational Operator2 : RelationalOperator  OutDataTypeStr=boolean
  LbDCC_FinishInStepChrg_flg : Outport
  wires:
  LcDCC_StepChrgCrntReq_A/1 -> Relational Operator/1
  Relational Operator1/1 -> BMSDebounceStartZero/1
  GcCDP_MaxCellVolt_mV/1 -> Relational Operator2/1, Relational Operator1/1
  Add/1 -> Relational Operator1/2
  Constant3/1 -> Add/2
  BMSDebounceStartZero/1 -> Logical Operator1/2
  Logical Operator1/1 -> LbDCC_FinishInStepChrg_flg/1  "LbDCC_FinishInStepChrg_flg"
  Constant/1 -> Relational Operator/2
  Constant2/1 -> BMSDebounceStartZero/3
  GcUDS_FullChrgCutoffVolt_mV/1 -> Relational Operator2/2, Add/1
  Relational Operator/1 -> Logical Operator2/1
  Relational Operator2/1 -> Logical Operator2/2
  Logical Operator2/1 -> BMSDebounceStartZero1/1
  BMSDebounceStartZero1/1 -> Logical Operator1/1
  Constant6/1 -> BMSDebounceStartZero1/3
  Constant1/1 -> BMSDebounceStartZero/4
  Constant8/1 -> BMSDebounceStartZero/5
  Constant9/1 -> BMSDebounceStartZero/2
  Constant7/1 -> BMSDebounceStartZero1/4
  Constant10/1 -> BMSDebounceStartZero1/5
  Constant11/1 -> BMSDebounceStartZero1/2

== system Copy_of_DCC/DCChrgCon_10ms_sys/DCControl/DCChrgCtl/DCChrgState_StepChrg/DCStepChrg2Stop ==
  LbDCC_FinishInStepChrg_flg : Inport
  GbDCC_DCChrgPrmt_flg : Inport  Port=2
  GeVDP_ChrgRqst_enum : Inport  Port=3
  GeDCC_DCConnSt_enum : Inport  Port=4
  Constant : Constant  Value=Enum_VDPChrgRqst.Enum_VDPChrgRqst_PowerDown
  Constant3 : Constant  Value=ASWTYPE_FALSE
  Constant9 : Constant  Value=Enum_DCCDCConnSt.Enum_DCCDCConnSt_Chrging
  Data Type Conversion1 : DataTypeConversion
  Data Type Conversion5 : DataTypeConversion
  Logical Operator1 : Logic  Operator=OR  Inputs=4  AllPortsSameDT=off  OutDataTypeStr=boolean
  Relational Operator1 : RelationalOperator  Operator===  OutDataTypeStr=boolean
  Relational Operator5 : RelationalOperator  Operator===  OutDataTypeStr=boolean
  Relational Operator8 : RelationalOperator  Operator=~=  OutDataTypeStr=boolean
  LbDCC_StepChrg2Stop_flg : Outport
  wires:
  GbDCC_DCChrgPrmt_flg/1 -> Relational Operator1/1
  Logical Operator1/1 -> LbDCC_StepChrg2Stop_flg/1  "LbDCC_StepChrg2Stop_flg"
  Relational Operator1/1 -> Logical Operator1/1
  Constant3/1 -> Relational Operator1/2
  LbDCC_FinishInStepChrg_flg/1 -> Logical Operator1/2
  GeVDP_ChrgRqst_enum/1 -> Data Type Conversion1/1
  Constant/1 -> Relational Operator5/2
  Data Type Conversion1/1 -> Relational Operator5/1
  Relational Operator5/1 -> Logical Operator1/3
  Constant9/1 -> Relational Operator8/2
  Data Type Conversion5/1 -> Relational Operator8/1
  GeDCC_DCConnSt_enum/1 -> Data Type Conversion5/1
  Relational Operator8/1 -> Logical Operator1/4

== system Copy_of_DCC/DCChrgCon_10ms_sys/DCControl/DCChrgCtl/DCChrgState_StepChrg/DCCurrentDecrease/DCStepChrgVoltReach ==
  LcDCC_LastCrntRqst_A : Inport
  Enable : EnablePort  StatesWhenEnabling=reset
  Add : Sum  Inputs=+-  AccumDataTypeStr=single  OutDataTypeStr=single
  BMSDelay : AIWAYS_Powertrain_BMS_lib/Debounce & Delay/BMSDelay
  Constant : Constant  Value=ASWTYPE_TRUE
  Constant2 : Constant  Value=DCC_RUNTIME_MS
  Constant3 : Constant  Value=CcDCC_DCChrgStepCurr_A
  Constant4 : Constant  Value=DCC_CONST0_NUMB
  Constant5 : Constant  Value=CcDCC_DCStepChrgWaitTime_ms
  Data Type Conversion : DataTypeConversion
  Limiter : AIWAYS_Powertrain_BMS_lib/Nonlinear Blocks/Limiter
  Switch : Switch  Criteria=u2 ~= 0
  LbDCC_DCStepWaitReach_flg : Outport
  LcDCC_StepChrgCrntDec_A : Outport  Port=2
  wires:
  BMSDelay/1 -> Switch/2, LbDCC_DCStepWaitReach_flg/1  "LbDCC_DCStepWaitReach_flg"
  LcDCC_LastCrntRqst_A/1 -> Limiter/1, Add/1, Switch/3
  Constant3/1 -> Add/2
  Add/1 -> Limiter/3
  Limiter/1 -> Switch/1
  Constant/1 -> BMSDelay/1
  Constant2/1 -> BMSDelay/2
  Constant5/1 -> BMSDelay/3
  Switch/1 -> LcDCC_StepChrgCrntDec_A/1  "LcDCC_StepChrgCrntDec_A"
  Constant4/1 -> Data Type Conversion/1
  Data Type Conversion/1 -> Limiter/2

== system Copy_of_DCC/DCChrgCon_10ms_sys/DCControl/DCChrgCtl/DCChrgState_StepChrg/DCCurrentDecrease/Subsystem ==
  GcDCC_DCChrgCrntRqst_A : Inport
  Enable : EnablePort
  Signal Conversion : SignalConversion  ConversionOutput=Contiguous copy  OverrideOpt=off
  LcDCC_DCChrgCrntRqstLock_A : Outport
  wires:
  GcDCC_DCChrgCrntRqst_A/1 -> Signal Conversion/1
  Signal Conversion/1 -> LcDCC_DCChrgCrntRqstLock_A/1
